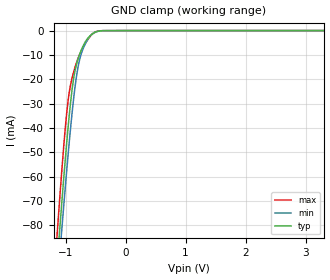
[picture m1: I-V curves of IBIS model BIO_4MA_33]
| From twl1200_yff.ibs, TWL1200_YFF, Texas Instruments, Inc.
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[Model]   BIO_4MA_33
Model_type  Input
Vinl=1.155
Vinh=2.145
| variable   typ   min   max
C_comp   2.71pF   2.25pF   3.45pF
[Temperature Range]   40   100   -40
| Ambient temperature   25   85   -40
[Voltage range]   3.3   3   3.6
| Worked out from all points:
|   GND clamp passes 1 mA (typ) near -0.53 V on its own axis
[GND Clamp]
| BIO_4MA_33
|   Voltage   I(typ)   I(min)   I(max)
-3.3V     -887.8mA   -863.1mA   -919.1mA
-1.15V    -99.03mA   -109.1mA   -87.2mA
-1.13V    -92.43mA   -102.7mA   -80.25mA
-1.1V     -82.67mA   -93.35mA   -70.01mA
-1.07V    -73.08mA   -84.08mA   -60.07mA
-960mV    -40.49mA   -51.77mA   -29.36mA
-895mV    -25.04mA   -34.79mA   -19.91mA
-845mV    -16.9mA    -23.75mA   -15.35mA
-790mV    -11.53mA   -14.76mA   -11.3mA
-730mV    -7.566mA   -8.933mA   -7.995mA
-505mV    -695.7uA   -602.4uA   -577.8uA
3.3V      791.9pA    1.015uA    126.9pA
